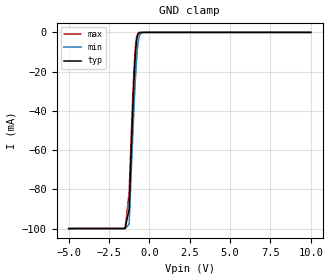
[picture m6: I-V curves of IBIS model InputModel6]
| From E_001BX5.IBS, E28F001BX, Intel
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|************************Input Model 6******************************
[Model]   InputModel6
Model_type   Input
|   Model for pins OE#, CE# and WE#
Vinl = 0.8V
Vinh = 2.0V
|Variable   Typ   Min   Max
C_comp   9.13p   7.20p   11.06p
[Voltage Range]   5.0V   4.5V   5.5V
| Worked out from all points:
|   GND clamp passes 1 mA (typ) near -0.71 V on its own axis
[GND_clamp]
|Voltage   I(typ)   I(min)   I(max)
-5V       -99.95mA   -99.95mA   -99.85mA
-1.5V     -99.85mA   -99.95mA   -99.85mA
-1.25V    -90.08mA   -97.62mA   -81.15mA
-1.05V    -44.14mA   -56.66mA   -37.31mA
-950mV    -24.34mA   -37.9mA    -18.84mA
-900mV    -16.1mA    -29.37mA   -11.47mA
-850mV    -9.617mA   -21.76mA   -6.09mA
-800mV    -4.899mA   -14.98mA   -2.617mA
-700mV    -799.9uA   -5.46mA    -294.2uA
-600mV    -85.03uA   -1.356mA   -30.51uA
-250mV    0A         0A         0A
10V       0A         0A         0A
[Power_clamp]
| Input buffer circuits of this product do not intrinisically
| require a [Power_clamp] defintion.  This zero current
| [Power_clamp] table is provided for compatibility with
| some IBIS parsers.
|Voltage   I(typ)   I(min)   I(max)
-5V       0A         0A         0A
0V        0A         0A         0A
5V        0A         0A         0A
10V       0A         0A         0A
